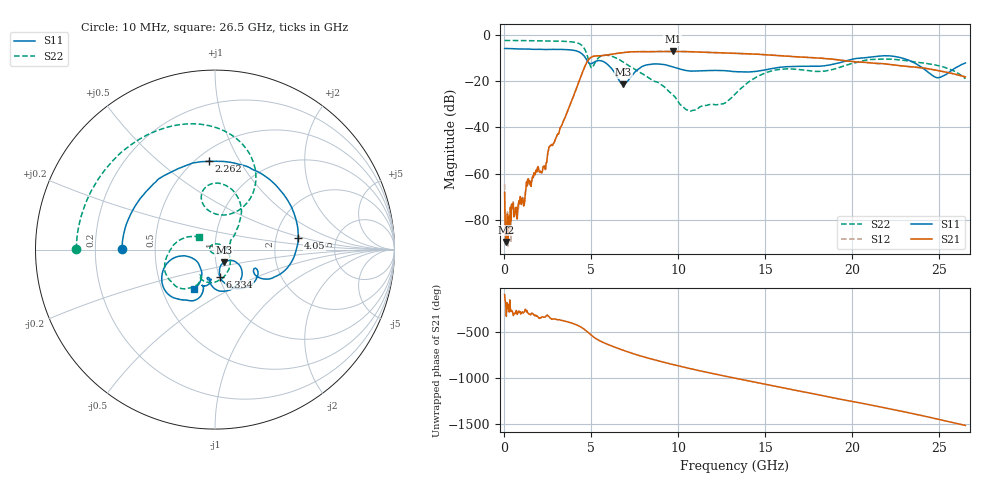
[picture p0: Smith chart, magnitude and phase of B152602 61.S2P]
!  2-Port S-parameters saved by WinCal
! VAR MeasName=S-Parameters (CALIBRATED_DATA) read from VNA (N5242A)
! VAR MeasDate=2016-1-5 16:34:32
! VAR NAME=B152602 61
! VAR FILENAME=B152602 61.S2P
! VAR DATE=2016-1-5 16:34:32
! VAR PHYS_PORTS=1,2
# Hz S DB R 50
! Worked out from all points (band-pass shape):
!   801 points, 10 MHz to 26.5 GHz, reference 50 ohm
!   highest |S21| = -7.00 dB at 9.679 GHz (marker M1); lowest = -89.7 dB at 109.3 MHz (marker M2)
!   |S21| within 3 dB of the highest: 4.902 GHz to 18.29 GHz (13.39 GHz wide, 115 % of centre)
!   lowest |S11| = -21.3 dB at 6.831 GHz (marker M3), VSWR 1.19, Z = 54.5 - j7.81 ohm
!   |S11| at or under -10 dB: 4.674 GHz to 20.29 GHz (15.61 GHz wide, 125 % of centre); 22.92 GHz to end of sweep
!   |S22| runs from -32.9 to -2.2 dB; largest |S21 - S12| = 0.0031
!   S11 on the Smith chart (normalised r, x): 10 MHz: 0.32, +0.00; 2.262 GHz: 0.58, +0.75; 4.05 GHz: 2.68, +0.44; 6.334 GHz: 1.01, -0.31; 26.5 GHz: 0.72, -0.34
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1e7  -5.73 179.6  -68.11 -100.4  -64.61 57.8  -2.23 179.8
1.093375e8  -5.72 175.8  -89.71 25.9  -89.17 -109.3  -2.24 178.3
2.417875e8  -5.74 170.6  -85.34 74.8  -86.86 129.5  -2.25 176.3
6.7225e8  -5.88 154.4  -74.65 88.6  -77.59 77.6  -2.27 169.6
1.367612e9  -5.95 128.8  -62.35 58.6  -62.79 63.5  -2.32 158.7
2.26165e9  -6.14 93.9  -57.12 15.3  -56.82 11.7  -2.42 143.6
4.049725e9  -6.59 7.8  -24.85 -59.9  -24.84 -60.0  -3.04 97.2
4.447075e9  -7.99 -18.3  -16.82 -96.8  -16.81 -96.6  -4.36 75.2
5.109325e9  -11.85 -24.9  -9.11 163.7  -9.10 163.8  -13.34 97.8
5.639125e9  -11.25 -49.6  -8.79 106.7  -8.77 106.8  -8.80 94.9
6.334488e9  -16.26 -79.1  -8.03 52.9  -8.01 53.0  -9.56 69.9
6.831175e9  -21.30 -55.7  -7.49 18.5  -7.48 18.7  -11.58 55.9
8.851038e9  -12.46 -74.9  -7.05 -95.4  -7.02 -95.4  -20.54 24.5
9.67885e9  -13.70 -94.0  -7.00 -134.6  -7.00 -134.6  -25.80 -10.0
1.070534e10  -15.53 -97.4  -7.13 179.9  -7.11 179.9  -32.91 -110.6
1.3255e10  -15.78 -104.9  -7.81 77.7  -7.79 77.7  -25.57 16.7
1.530798e10  -14.51 -99.3  -8.56 -0.5  -8.53 -0.4  -15.56 -77.3
1.769208e10  -13.47 -109.6  -9.70 -88.1  -9.66 -87.9  -15.55 -120.8
1.971194e10  -10.95 -108.4  -11.15 -163.2  -11.11 -163.5  -12.82 -118.4
2.209604e10  -8.89 -141.3  -12.63 109.1  -12.56 108.7  -10.31 -153.8
2.487749e10  -18.43 -145.4  -15.24 -2.6  -15.24 -2.4  -13.06 170.7
2.65e10  -12.00 -118.2  -18.05 -71.8  -18.02 -71.9  -18.84 142.5
